(* Logix 5000 DataType export Std_DiscreteAlarm; software revision 30.00 *)

TYPE Std_DiscreteAlarm :   // ALARM RESET
STRUCT
   AckC : BOOL;   // ALARM ACKNOWLEDGE
   LatchA : BOOL;   // ALARM LATCH
   DetectS : BOOL;   // ALARM DETECT
   BitS : BOOL;   // ALARM MISCOMPARE
   InhibitC : BOOL;   // ALARM INHIBIT
   Tmr : TIMER;   // ALARM Timer
END_STRUCT
END_TYPE
